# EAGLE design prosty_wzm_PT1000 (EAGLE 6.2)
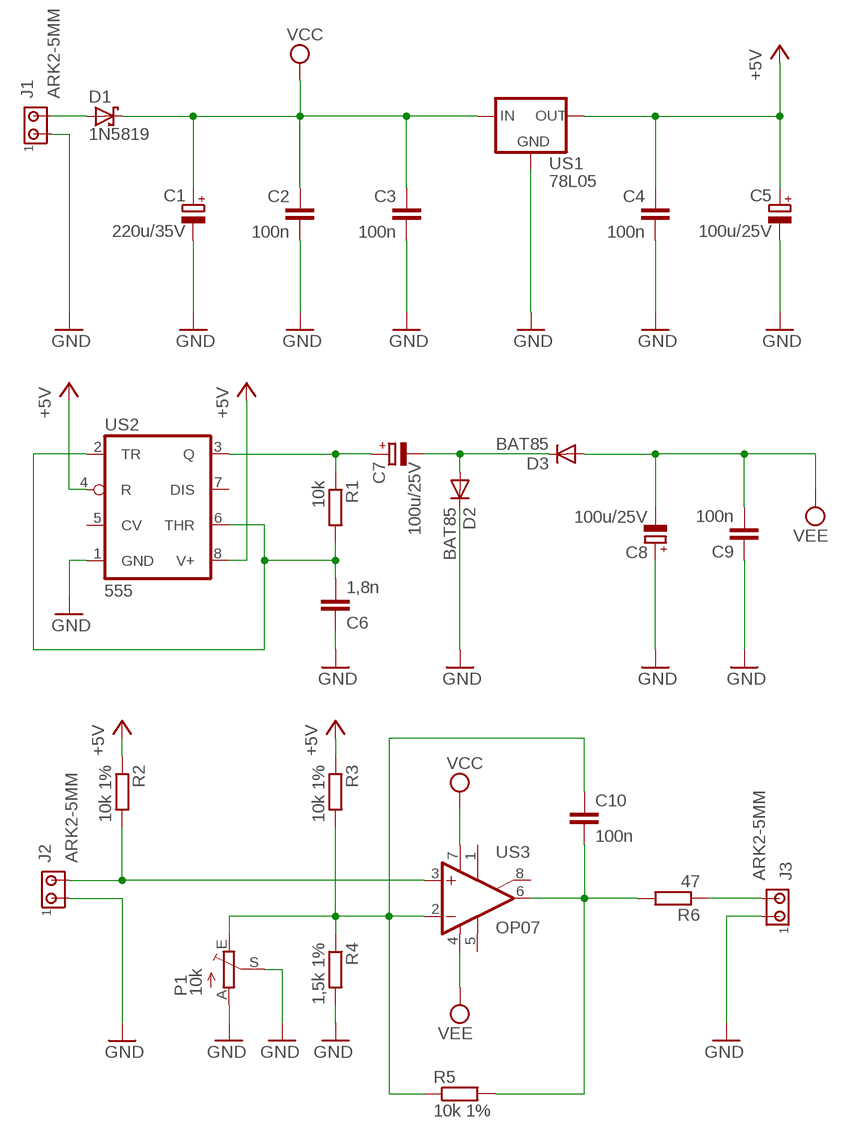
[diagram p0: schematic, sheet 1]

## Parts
C1  220u/35V  CPOL-EUE3.5-8  [E3,5-8]
C2  100n  C-EU050-025X075  [C050-025X075]
C3  100n  C-EU050-025X075  [C050-025X075]
C4  100n  C-EU050-025X075  [C050-025X075]
C5  100u/25V  CPOL-EUE2.5-6  [E2,5-6]
C6  1,8n  C-EU050-025X075  [C050-025X075]
C7  100u/25V  CPOL-EUE2.5-6  [E2,5-6]
C8  100u/25V  CPOL-EUE2.5-6  [E2,5-6]
C9  100n  C-EU050-025X075  [C050-025X075]
C10  100n  C-EU050-025X075  [C050-025X075]
D1  1N5819  1N5819-T  [DO41-7.6]
D2  BAT85  BAT81  [DO34-7]
D3  BAT85  BAT81  [DO34-7]
J1  ARK2-5MM  [2PIN-5MM]
J2  ARK2-5MM  [2PIN-5MM]
J3  ARK2-5MM  [2PIN-5MM]
P1  10k  TRIM_EU-B64Y  [B64Y]
R1  10k  R-EU_0207/7  [0207/7]
R2  10k 1%  R-EU_0207/7  [0207/7]
R3  10k 1%  R-EU_0207/7  [0207/7]
R4  1,5k 1%  R-EU_0207/7  [0207/7]
R5  10k 1%  R-EU_0207/7  [0207/7]
R6  47  R-EU_0207/7  [0207/7]
US1  78L05  78LXX  [78LXX]
US2  555  LM555N  [DIL08]
US3  OP07  OP07CN  [DIL08]

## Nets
+5V: C4.1 C5.+ R2.1 R3.1 US1.OUT US2.4(R) US2.8(V+)
GND: C1.- C2.2 C3.2 C4.2 C5.- C6.1 C8.+ C9.1 D2.C J1.P$1 J2.P$1 J3.P$1 P1.A P1.S R4.2 US1.GND US2.1(GND)
N$1: C7.+ R1.1 US2.3(Q)
N$2: C7.- D2.A D3.C
N$3: C6.2 R1.2 US2.2(TR) US2.6(THR)
N$4: D1.A J1.P$2
N$5: C10.2 R5.2 R6.2 US3.6(OUT)
N$6: C10.1 P1.E R3.2 R4.1 R5.1 US3.2(-IN)
N$7: J2.P$2 R2.2 US3.3(+IN)
N$11: J3.P$2 R6.1
VCC: C1.+ C2.1 C3.1 D1.C US1.IN US3.7(V+)
VEE: C8.- C9.2 D3.A US3.4(V-)
Unconnected: US2.5(CV) US2.7(DIS) US3.1(ON1) US3.5(OPT) US3.8(ON2)

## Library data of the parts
C1 C5 C7 C8 = rcl:CPOL-EU: POLARIZED CAPACITOR, European symbol
C2-C4 C6 C9 C10 = rcl:C-EU: CAPACITOR, European symbol
D1 = diode:1N581*: 1.0A SCHOTTKY BARRIER RECTIFIER
D2 D3 = diode:BAT81: DIODE
J1-J3 = zlacza_futrzak:ARK2: ARK 2
P1 = pot:TRIM_EU-: POTENTIOMETER
R1-R6 = rcl:R-EU_: RESISTOR, European symbol
US1 = v-reg:78LXX: VOLTAGE REGULATOR
US2 = linear:*555: TIMER
US3 = linear:OP07*: OP AMP

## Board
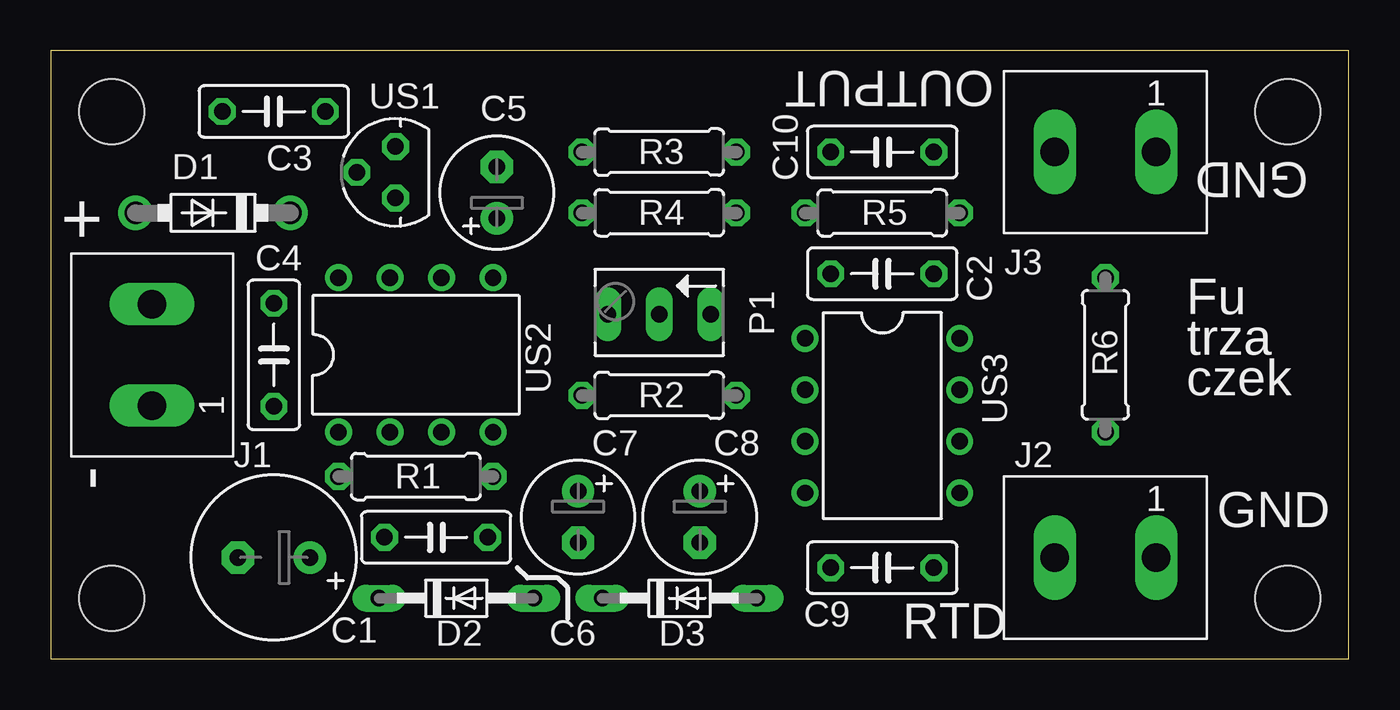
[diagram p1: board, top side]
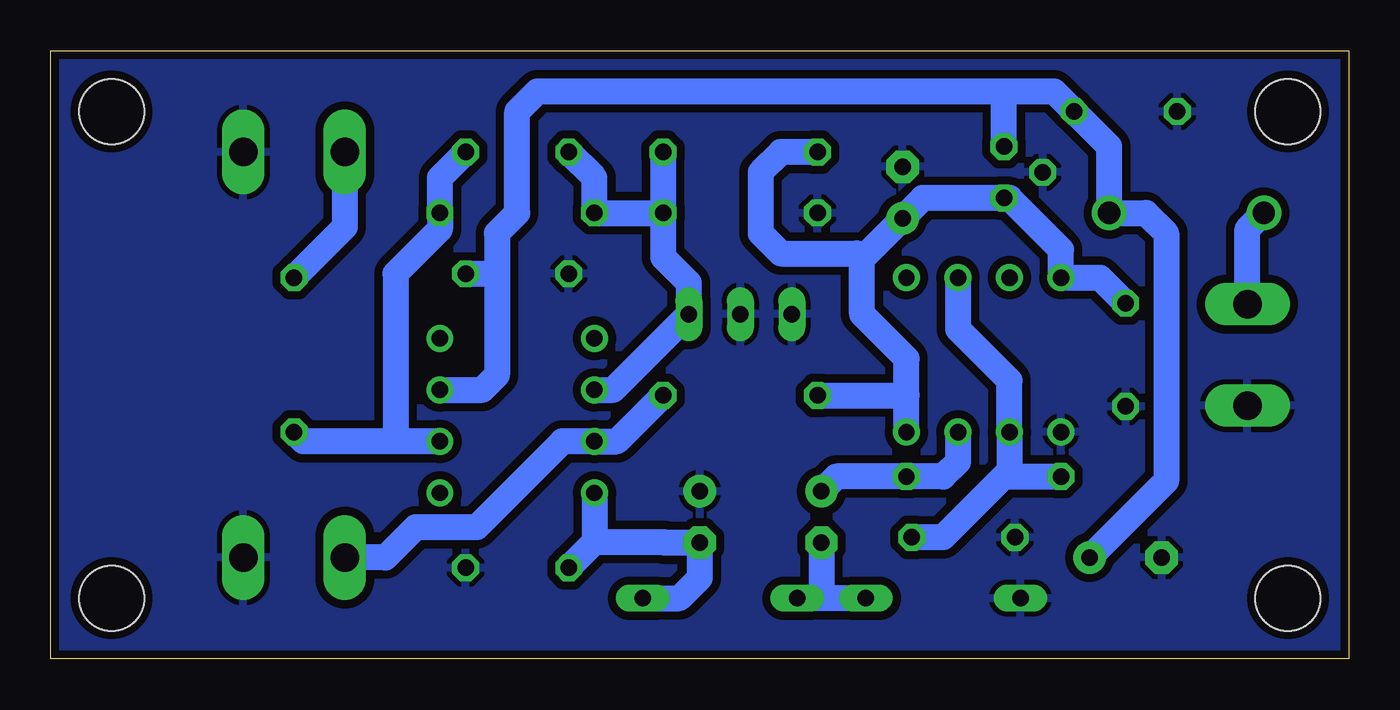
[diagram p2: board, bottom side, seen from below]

Size 64 x 30 mm. Coordinates in mm from the lower left corner, seen from the top.
Outline: 0,0 64,0 64,30 0,30 0,0
Copper layers (1*16): Top 0.035mm / dielectric 1.5mm / Bottom 0.035mm
Design rules: minimum track width 10mil, minimum drill 24mil, track to track 8mil, track to pad 8mil, pad to pad 8mil, via to via 8mil, smd to smd 8mil, copper to edge 15mil, drill to drill 8mil, minimum pad ring 10mil, minimum via ring 8mil, stop-mask expansion 4mil, vias tented up to drill 0mil, thermal gap 10mil
Holes 3.2 mm at 3,3 3,27 61,3 61,27

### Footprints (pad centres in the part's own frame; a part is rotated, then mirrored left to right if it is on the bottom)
E3,5-8 = drill 0.813 pad 1.6: + -1.778,0 | drill 0.813 pad 1.6 octagon: - 1.778,0
C050-025X075 = drill 0.813 octagon: 1 -2.54,0; 2 2.54,0
E2,5-6 = drill 0.813 pad 1.6: + -1.27,0 | drill 0.813 pad 1.6 octagon: - 1.27,0
DO41-7.6 = drill 1.1 pad 1.7: A 3.81,0; C -3.81,0
DO34-7 = drill 0.813 long: A 3.81,0; C -3.81,0
2PIN-5MM = drill 1.4 long: P$1 -2.5,0; P$2 2.5,0
B64Y = drill 0.813 long: A 2.54,0; E -2.54,0; S 0,0
0207/7 = drill 0.813 octagon: 1 -3.81,0; 2 3.81,0
78LXX = drill 0.813 octagon: GND 0,1.905; IN 1.27,0; OUT -1.27,0
DIL08 = drill 0.813 pad 1.27: 1 -3.81,-3.81; 2 -1.27,-3.81; 3 1.27,-3.81; 4 3.81,-3.81; 5 3.81,3.81; 6 1.27,3.81; 7 -1.27,3.81; 8 -3.81,3.81

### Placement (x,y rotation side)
C1  11,5 180 top
C2  41,19 180 top
C3  11,27 180 top
C4  11,15 270 top
C5  22,23 90 top
C6  19,6 0 top
C7  26,7 270 top
C8  32,7 270 top
C9  41,4.5 180 top
C10  41,25 0 top
D1  8,22 180 top
D2  20,3 0 top
D3  31,3 0 top
J1  5,15 90 top
J2  52,5 180 top
J3  52,25 180 top
P1  30,17 180 top
R1  18,9 180 top
R2  30,13 0 top
R3  30,25 0 top
R4  30,22 180 top
R5  41,22 0 top
R6  52,15 270 top
US1  17,24 90 top
US2  18,15 0 top
US3  41,12 270 top

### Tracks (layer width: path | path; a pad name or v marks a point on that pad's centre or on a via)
+5V
  Bottom 1.27: C4.1 12.27,18.81 US2.8 14.19,20.19 16.73,22.73 US1.OUT 21,22.73 C5.+ 24,19.73 | US2.4 21.81,13 | 21.81,13 21.81,14.81 24,17 24,19.73 | R2.1 21.81,13 | R3.1 28,25 29,24 29,21 28,20 24.27,20 24,19.73
GND
  pour Bottom (isolate 0.406): 0,30 64,30 64,0 0,0
N$1
  Bottom 1.27: US2.3 19.27,9.73 20,9 R1.1 25.27,9 C7.+
N$2
  Bottom 1.27: D2.A 26,3 | 26,3 D3.C | C7.- 26,3
N$3
  Bottom 1.27: 17,9 R1.2 | 17,9 20,6 C6.2 | 17,9 16.73,9.27 US2.2 16.73,13.73 19.27,16.27 US2.6
N$4
  Bottom 1.27: J1.P$2 5,21.19 D1.A
N$5
  Bottom 1.27: C10.2 44.81,23.73 R5.2 44.81,21.19 47,19 47,10.73 | US3.6 47,10.73 | 47,10.73 51.54,10.73 R6.2
N$6
  Bottom 1.27: R3.2 R4.1 | R4.1 33.81,19.81 32.54,18.54 P1.E 36.27,13.27 US3.2 | R4.1 R5.1 37.19,23.73 C10.1
N$7
  Bottom 1.27: R2.2 36.08,10.73 US3.3 38.77,10.73 43,6.5 46,6.5 47.5,5 J2.P$2
N$11
  Bottom 1.27: J3.P$2 49.5,21.31 R6.1
VCC
  Bottom 1.27: C1.+ 9,8.78 9,21 10,22 D1.C 11.81,25.27 C3.1 14.54,28 17,28 | 42,19 42,21 41,22 41,27 40,28 17,28 | 42,19 42,14 42.73,13.27 US3.7 | US1.IN 17,28 | C2.1 42,19
VEE
  Bottom 1.27: D3.A 33,3 32,4 C8.- 33.73,5.73 33.77,5.77 37.19,5.77 | US3.4 37.19,5.77 | 37.19,5.77 C9.2

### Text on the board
tPlace: OUTPUT | GND | + | Fu | trza | czek | - | GND | RTD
